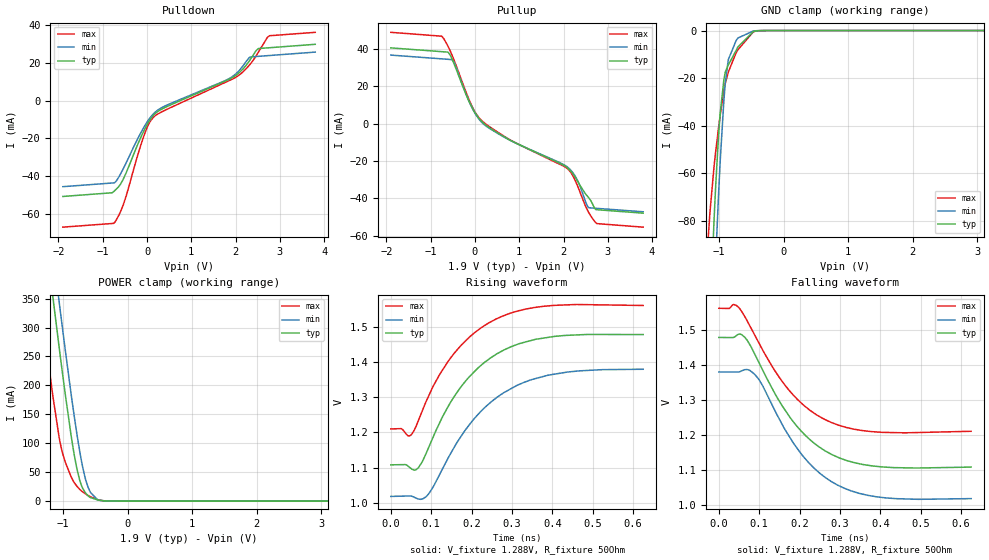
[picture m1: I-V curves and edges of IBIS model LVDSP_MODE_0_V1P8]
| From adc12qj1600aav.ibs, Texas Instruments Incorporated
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[Model]   LVDSP_MODE_0_V1P8
Model_type   3-state
Polarity   Non-Inverting
Vmeas = 1.3
Vref = 1.3
Cref = 0.2pF
Rref = 50
|   typ   min   max
C_comp   1.95pF   1.92pF   1.97pF
[Voltage Range]   1.9   1.8   2
[Temperature Range]   25   125   -40
[Pullup Reference]   1.9   1.8   2
[Pulldown Reference]   0   0   0
[Power Clamp Reference]   1.9   1.8   2
[GND Clamp Reference]   0   0   0
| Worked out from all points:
|   slope of the pulldown table from 0 to 0.285 V, typ, clamps not added: 37.5 ohm
|   slope of the pullup table from 0 to 0.285 V, typ, clamps not added: 38.4 ohm
|   GND clamp passes 1 mA (typ) near -0.49 V on its own axis
|   POWER clamp passes 1 mA (typ) near -0.40 V on its own axis
|   falling waveform, V_fixture 1.288V, R_fixture 50Ohm: 20-80 % time 130ps typ, 128ps min, 129ps max; typ from 1.48 V to 1.11 V
|   rising waveform, V_fixture 1.288V, R_fixture 50Ohm: 20-80 % time 135ps typ, 147ps min, 131ps max; typ from 1.11 V to 1.48 V
[Pulldown]
|   Voltage   I(typ)   I(min)   I(max)
-1.9V     -50.94mA   -45.74mA   -67.23mA
-731.5mV  -47.88mA   -43.61mA   -64.74mA
-537.7mV  -41.82mA   -36.27mA   -55.46mA
-150.1mV  -20.08mA   -17.58mA   -24.37mA
-24.7mV   -13.93mA   -12.39mA   -15.9mA
180.5mV   -7.046mA   -6.267mA   -8.179mA
1.765V    10.33mA    10.57mA    9.605mA
2.067V    14.5mA     15.54mA    13.26mA
2.329V    21.63mA    23.07mA    19.29mA
2.518V    27.58mA    23.45mA    25.78mA
2.768V    28.03mA    23.89mA    34.39mA
3.8V      29.84mA    25.7mA     36.2mA
[GND Clamp]
|   Voltage   I(typ)   I(min)   I(max)
-1.9V     -792mA     -835.5mA   -701.6mA
-1.182V   -151mA     -191.9mA   -93.04mA
-1.142V   -121.8mA   -160.8mA   -76.76mA
-1.079V   -80.7mA    -115mA     -57.63mA
-1.051V   -64.59mA   -95.69mA   -50.6mA
-1.011V   -45.56mA   -70.81mA   -41.59mA
-982.3mV  -34.83mA   -54.95mA   -35.62mA
-902.5mV  -17.4mA    -21.83mA   -22.1mA
-856.9mV  -14.48mA   -12.24mA   -17.5mA
-708.7mV  -6.916mA   -3.174mA   -8.113mA
-383.8mV  -88.23uA   -45.04uA   -73.67uA
3.8V      0A         0A         0A
[Pullup]
|   Voltage   I(typ)   I(min)   I(max)
-1.9V     40.49mA    36.64mA    48.82mA
-748.6mV  38.47mA    34.62mA    46.67mA
-606.1mV  38.15mA    34.37mA    41.23mA
-497.8mV  33.49mA    33.72mA    35.44mA
-98.8mV   10.22mA    9.995mA    10.9mA
163.4mV   830.7uA    400.5uA    1.34mA
807.5mV   -9.049mA   -9.164mA   -8.915mA
2.084V    -23.58mA   -23.18mA   -24.04mA
2.307V    -30.4mA    -29.98mA   -32.74mA
2.557V    -39.36mA   -44.82mA   -47.09mA
2.751V    -46.12mA   -45.38mA   -53.54mA
3.8V      -47.96mA   -47.22mA   -55.45mA
[POWER Clamp]
|   Voltage   I(typ)   I(min)   I(max)
-1.9V     1.054A     1.134A     877.8mA
-1.313V   493.9mA    574mA      316.4mA
-1.159V   352.1mA    431.6mA    180.8mA
-1.062V   265.4mA    344mA      109.7mA
-970.9mV  187.3mA    263.8mA    68.47mA
-868.3mV  107mA      177.9mA    39.97mA
-788.5mV  56.31mA    116.7mA    25.87mA
-697.3mV  22.01mA    58.3mA     15.96mA
-577.6mV  6.145mA    15.02mA    7.549mA
-469.3mV  2.173mA    2.573mA    2.732mA
-315.4mV  277.1uA    170.5uA    214.9uA
3.8V      0A         0A         0A
[Ramp]
R_load = 50
|   typ   min   max
dV/dt_r   0.222231/1.35034e-10   0.216971/1.46981e-10   0.210551/1.31224e-10
dV/dt_f   0.221877/1.29539e-10   0.216787/1.27496e-10   0.210551/1.28486e-10
[Falling Waveform]
V_fixture = 1.288V
V_fixture_min = 1.185V
V_fixture_max = 1.389V
R_fixture = 50Ohm
C_fixture = 0F
|   Time   V(typ)   V(min)   V(max)
0s        1.478V     1.379V     1.561V
43.08ps   1.483V     1.379V     1.569V
64.02ps   1.479V     1.386V     1.538V
89.03ps   1.43V      1.372V     1.485V
176.3ps   1.25V      1.192V     1.324V
211.5ps   1.202V     1.135V     1.283V
259.6ps   1.157V     1.082V     1.245V
311.1ps   1.129V     1.048V     1.223V
389.6ps   1.11V      1.023V     1.208V
625ps     1.108V     1.018V     1.21V
[Rising Waveform]
V_fixture = 1.288V
V_fixture_min = 1.185V
V_fixture_max = 1.389V
R_fixture = 50Ohm
C_fixture = 0F
|   Time   V(typ)   V(min)   V(max)
0s        1.108V     1.018V     1.21V
50.37ps   1.097V     1.019V     1.193V
66.96ps   1.098V     1.011V     1.23V
87.18ps   1.14V      1.017V     1.288V
121ps     1.228V     1.081V     1.365V
168.9ps   1.322V     1.18V      1.441V
211.5ps   1.378V     1.246V     1.487V
259.6ps   1.421V     1.297V     1.522V
389.6ps   1.47V      1.363V     1.56V
625ps     1.478V     1.38V      1.561V
